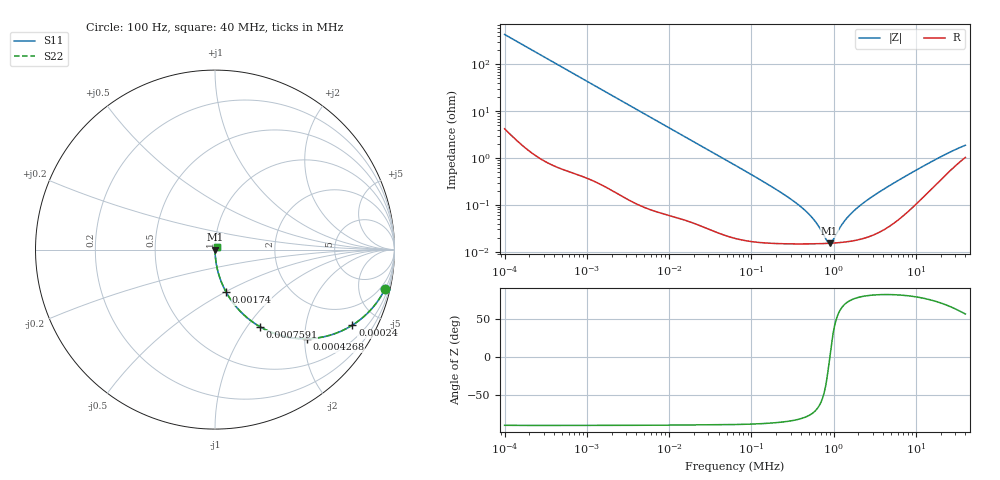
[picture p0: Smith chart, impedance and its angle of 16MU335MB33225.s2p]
!Components F PML CAP
!CONCATENATE F 0.1-40000kHz, at 20deg DC=0V
!Part Number F 16MU335MB33225
!Copyright(C) Rubycon Corporation. 20161128
# MHz S MA R 50
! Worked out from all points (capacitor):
!   561 points, 100 Hz to 40 MHz, reference 50 ohm
!   read as one part in series: C = 3.66 uF near 104.7 Hz
!   lowest |Z| = 15.2 mohm at 894.2 kHz (marker M1)
!   series resonance near 898.3 kHz, so ESL is about 8.6 nH
!   S11 on the Smith chart (normalised r, x): 100 Hz: 1.08, -8.70; 240 Hz: 1.02, -3.63; 426.8 Hz: 1.01, -2.04; 759.1 Hz: 1.01, -1.15; 1.74 kHz: 1.00, -0.50; 40 MHz: 1.02, +0.03
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0.0001  0.9725 -12.9  0.2235 76.5  0.2235 76.5  0.9725 -12.9
0.0001585162  0.9374 -20.0  0.3415 69.6  0.3415 69.6  0.9374 -20.0
0.0002399605  0.8734 -28.8  0.4816 60.9  0.4816 60.9  0.8734 -28.8
0.0004268072  0.712 -44.2  0.6977 45.4  0.6977 45.4  0.712 -44.2
0.0007591432  0.4967 -59.8  0.8641 29.8  0.8641 29.8  0.4967 -59.8
0.0008716573  0.4465 -63.0  0.8912 26.5  0.8912 26.5  0.4465 -63.0
0.001739627  0.244 -75.3  0.9675 14.1  0.9675 14.1  0.244 -75.3
0.007424854  0.05934 -85.9  0.9975 3.4  0.9975 3.4  0.05934 -85.9
0.06324555  0.007073 -88.0  0.9998 0.4  0.9998 0.4  0.007073 -88.0
0.2762266  0.001484 -84.2  0.9999 0.1  0.9999 0.1  0.001484 -84.2
0.4086278  0.0008866 -80.4  0.9999 0.1  0.9999 0.1  0.0008866 -80.4
0.5512845  0.0005319 -73.8  0.9999 0.0  0.9999 0.0  0.0005319 -73.8
0.6628347  0.0003435 -64.3  0.9999 0.0  0.9999 0.0  0.0003435 -64.3
0.8345301  0.0001687 -26.4  0.9998 0.0  0.9998 0.0  0.0001687 -26.4
0.8942378  0.000152 -1.4  0.9998 0.0  0.9998 0.0  0.000152 -1.4
0.9805455  0.000175 28.8  0.9998 -0.0  0.9998 -0.0  0.000175 28.8
1.322865  0.000429 68.0  0.9998 -0.0  0.9998 -0.0  0.000429 68.0
1.704339  0.0007098 76.0  0.9998 -0.0  0.9998 -0.0  0.0007098 76.0
2.580015  0.001281 80.7  0.9998 -0.1  0.9998 -0.1  0.001281 80.7
4.69589  0.002531 82.1  0.9997 -0.1  0.9997 -0.1  0.002531 82.1
16.28983  0.008778 73.7  0.9976 -0.5  0.9976 -0.5  0.008778 73.8
40  0.01868 55.9  0.9896 -0.9  0.9896 -0.9  0.01868 55.9
